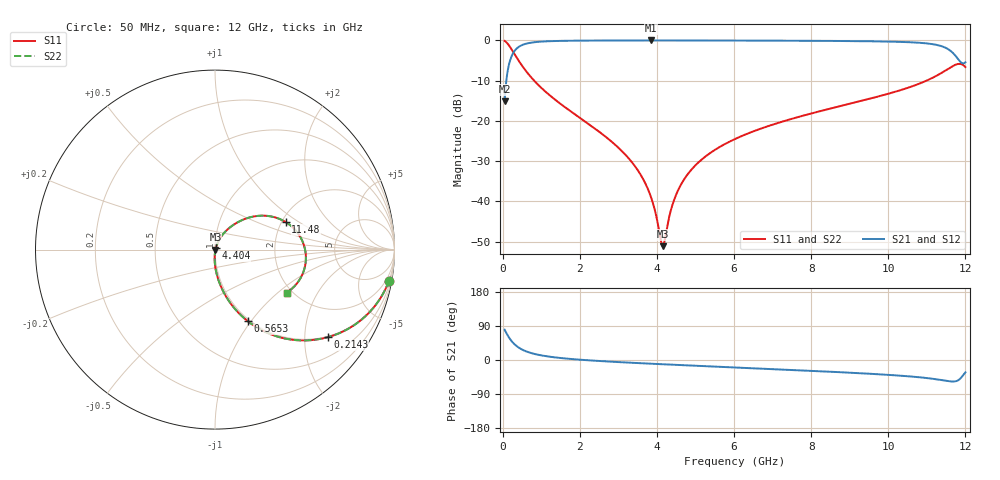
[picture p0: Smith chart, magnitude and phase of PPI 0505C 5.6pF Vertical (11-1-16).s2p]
# GHz S MA R 50
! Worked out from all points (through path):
!   1601 points, 50 MHz to 12 GHz, reference 50 ohm
!   highest |S21| = -0.03 dB at 3.837 GHz (marker M1); lowest = -15.2 dB at 50 MHz (marker M2)
!   group delay of S21, straight-line fit = 17 ps
!   lowest |S11| = -51.1 dB at 4.15 GHz (marker M3), VSWR 1.01, Z = 50.3 - j0.0588 ohm
!   |S11| at or under -10 dB: 815.2 MHz to 11 GHz (10.18 GHz wide, 172 % of centre)
!   |S22| runs from -51.1 to -0.1 dB; largest |S21 - S12| = 0
!   S11 on the Smith chart (normalised r, x): 50 MHz: 1, -11; 214.3 MHz: 0.98, -2.59; 565.3 MHz: 0.98, -0.97; 4.404 GHz: 1.01, +0.02; 11.48 GHz: 2.10, +0.79; 12 GHz: 1.87, -1.14
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0.05  0.9847 -10.2  0.1744 79.8  0.1744 79.8  0.9847 -10.2
0.139625  0.896 -26.7  0.4436 63.3  0.4436 63.3  0.896 -26.7
0.2143125  0.7955 -37.8  0.6054 52.1  0.6054 52.1  0.7955 -37.8
0.378625  0.5944 -54.5  0.8034 35.4  0.8034 35.4  0.5944 -54.5
0.5653438  0.4401 -65.3  0.8969 24.6  0.8969 24.6  0.4401 -65.3
1.043344  0.2463 -78.2  0.9677 11.4  0.9677 11.4  0.2463 -78.2
2.044156  0.1055 -88.4  0.9923 0.5  0.9923 0.5  0.1055 -88.4
3.231688  0.03579 -92.8  0.9967 -6.7  0.9967 -6.7  0.03579 -92.8
3.582719  0.02122 -91.6  0.997 -8.5  0.997 -8.5  0.02122 -91.6
3.836656  0.01164 -86.5  0.997 -9.8  0.997 -9.8  0.01164 -86.5
4.038312  0.004839 -66.3  0.997 -10.7  0.997 -10.7  0.004839 -66.3
4.150344  0.002774 -12.2  0.997 -11.3  0.997 -11.3  0.002774 -12.2
4.404281  0.009094 59.2  0.9968 -12.4  0.9968 -12.4  0.009094 59.2
4.635813  0.01653 66.2  0.9966 -13.5  0.9966 -13.5  0.01653 66.2
4.964437  0.02695 68.5  0.9962 -15.0  0.9962 -15.0  0.02695 68.5
6.025  0.05946 67.0  0.9944 -19.7  0.9944 -19.7  0.05946 67.0
8.019156  0.1241 59.2  0.987 -28.7  0.987 -28.7  0.1241 59.2
10.01331  0.218 48.0  0.9651 -39.3  0.9651 -39.3  0.218 48.0
10.91703  0.3046 38.1  0.9245 -46.7  0.9245 -46.7  0.3046 38.1
11.48466  0.4227 21.3  0.8091 -54.7  0.8091 -54.7  0.4227 21.3
11.79834  0.5074 -4.0  0.5958 -54.3  0.5958 -54.3  0.5074 -4.0
12  0.4653 -31.0  0.534 -32.5  0.534 -32.5  0.4653 -31.0
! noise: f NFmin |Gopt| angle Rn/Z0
0.05  0.0005408  0.9082  1.769  0.001294
1.372  0.004822  0.723  4.299  0.003448
2.701  0.007879  0.6755  7.621  0.004663
4.031  0.01064  0.6481  10.96  0.00569
5.36  0.01336  0.6319  14.25  0.006719
6.682  0.01625  0.6255  17.49  0.007941
8.012  0.01985  0.6327  20.74  0.009848
9.341  0.02603  0.668  24.1  0.01443
10.67  0.0462  0.7739  27.85  0.03936
12  0.316  0.9591  31.78  1.614
